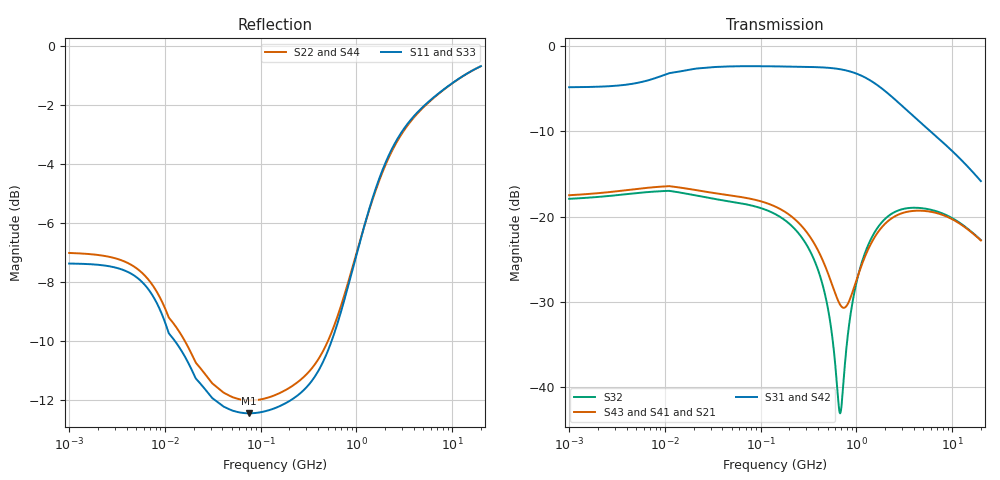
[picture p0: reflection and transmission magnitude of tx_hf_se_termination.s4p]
! Created Wed Jul 29 12:27:43 2015
# hz S db R 50
! 4 Port Network Data from SP1.SP block
! freq  dbS11  angS11  dbS12  angS12  dbS13  angS13  dbS14  angS14
!  dbS21  angS21  dbS22  angS22  dbS23  angS23  dbS24  angS24
!  dbS31  angS31  dbS32  angS32  dbS33  angS33  dbS34  angS34
!  dbS41  angS41  dbS42  angS42  dbS43  angS43  dbS44  angS44
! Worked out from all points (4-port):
!   861 points, 1 MHz to 20 GHz, reference 50 ohm
!   strongest paths, dB at 1 MHz, 11.89 MHz, 141.4 MHz, 1.682 GHz, 20 GHz:
!     S31: -4.8, -3.1, -2.4, -4.6, -15.8
!     S42: -5.1, -3.4, -2.5, -4.8, -15.8
!     S43: -17.5, -16.5, -18.8, -21.8, -22.8
!     S41: -17.5, -16.5, -18.8, -21.8, -22.8
!     S21: -17.5, -16.5, -18.8, -21.8, -22.8
!     S32: -17.9, -17.0, -19.7, -21.2, -22.7
!   lowest |S11| = -12.5 dB at 75.94 MHz (marker M1), VSWR 1.63, Z = 30.7 - j0.174 ohm
!   |S11| at or under -10 dB: 12.74 MHz to 551.9 MHz (539.2 MHz wide, 191 % of centre)
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1000000  -7.38 177.0  -17.91 1.5  -4.83 2.3  -17.91 1.5
         -17.49 1.7  -7.02 177.2  -17.49 1.7  -5.11 2.2
         -4.83 2.3  -17.91 1.5  -7.38 177.0  -17.91 1.5
         -17.49 1.7  -5.11 2.2  -17.49 1.7  -7.02 177.2
7.593646e7  -12.45 -179.4  -18.63 -18.5  -2.37 -0.2  -18.63 -18.5
            -17.87 -15.3  -12.01 -179.8  -17.87 -15.3  -2.51 -0.1
            -2.37 -0.2  -18.63 -18.5  -12.45 -179.4  -18.63 -18.5
            -17.87 -15.3  -2.51 -0.1  -17.87 -15.3  -12.01 -179.8
3.512446e8  -11.31 -158.8  -24.70 -53.4  -2.47 -7.5  -24.70 -53.4
            -22.87 -38.9  -10.88 -160.3  -22.87 -38.9  -2.65 -7.5
            -2.47 -7.5  -24.70 -53.4  -11.31 -158.8  -24.70 -53.4
            -22.87 -38.9  -2.65 -7.5  -22.87 -38.9  -10.88 -160.3
6.771391e8  -9.11 -147.1  -43.04 1.8  -2.72 -15.1  -43.04 1.8
            -30.31 -14.8  -8.90 -149.4  -30.31 -14.8  -2.92 -14.8
            -2.72 -15.1  -43.04 1.8  -9.11 -147.1  -43.04 1.8
            -30.31 -14.8  -2.92 -14.8  -30.31 -14.8  -8.90 -149.4
9.901874e8  -7.15 -144.6  -28.00 62.9  -3.21 -21.6  -28.00 62.9
            -27.63 30.0  -7.10 -146.6  -27.63 30.0  -3.39 -21.1
            -3.21 -21.6  -28.00 62.9  -7.15 -144.6  -28.00 62.9
            -27.63 30.0  -3.39 -21.1  -27.63 30.0  -7.10 -146.6
1.822976e9  -4.31 -149.5  -20.73 36.8  -4.93 -33.0  -20.73 36.8
            -21.31 26.6  -4.38 -150.5  -21.31 26.6  -5.04 -32.1
            -4.93 -33.0  -20.73 36.8  -4.31 -149.5  -20.73 36.8
            -21.31 26.6  -5.04 -32.1  -21.31 26.6  -4.38 -150.5
2e10  -0.69 -171.5  -22.74 -39.5  -15.83 -57.7  -22.74 -39.5
      -22.78 -39.4  -0.69 -171.5  -22.78 -39.4  -15.83 -57.7
      -15.83 -57.7  -22.74 -39.5  -0.69 -171.5  -22.74 -39.5
      -22.78 -39.4  -15.83 -57.7  -22.78 -39.4  -0.69 -171.5
